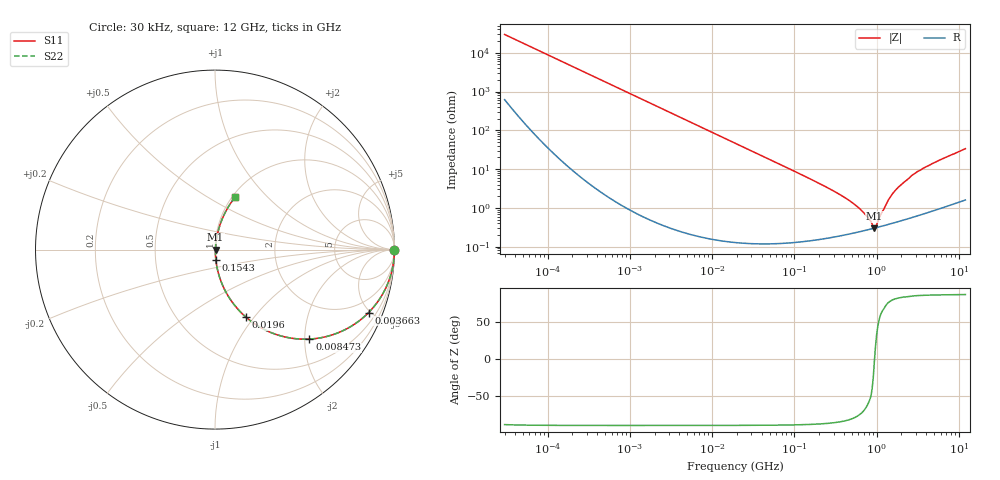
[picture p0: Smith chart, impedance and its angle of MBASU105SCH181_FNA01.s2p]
! MBASU105SCH181_FNA01  S-PARAMETER MODEL  ( General Type )
! Model Generated by TAIYO YUDEN Corporation (http://www.ty-top.com)
! Version 1.0
! TAIYO YUDEN Control No. 130207
! Copyright(c) 2013 TAIYO YUDEN CO.,LTD. All Rights Reserved.
! Product Description (link to TY-COMPAS)
! https://ds.yuden.co.jp/TYCOMPAS/or/detail?pn=MBASU105SCH181JFNA01&u=M
! Products Name : Multilayer Ceramic Capacitors
! Characteristics :
!  Capacitance : 180 pF , Rated Voltage : 50V , TCC : CH / C0H
!  Case Size : 1.0 x 0.5 / 0.039 x 0.02 [mm/inch] , Thickness : 0.5 / 0.02 [mm/inch]
!  (Conditions: Temperature = 25 degC , DC Bias Current/Voltage = 0A / 0V)
! External Node Assignments :
!  1  o---| |---o  2
! GND o---------o GND
! Frequency Range : 30000Hz  -  12GHz  [ 401 STEP ]
# MHz S RI R 50
! Freq[MHz].  S11 Real  S11 Imag  S21 Real  S21 Imag  S12 Real  S12 Imag  S22 Real  S22 Imag
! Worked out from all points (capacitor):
!   401 points, 30 kHz to 12 GHz, reference 50 ohm
!   read as one part in series: C = 178 pF near 32 kHz
!   lowest |Z| = 301 mohm at 939.2 MHz (marker M1)
!   series resonance near 943.3 MHz, so ESL is about 160 pH
!   S11 on the Smith chart (normalised r, x): 30 kHz: open; 3.663 MHz: 1.01, -4.87; 8.473 MHz: 1.00, -2.11; 19.6 MHz: 1.00, -0.91; 154.3 MHz: 1.00, -0.11; 12 GHz: 1.03, +0.67
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0.03  0.9999 -0.00336  8.15e-05 0.00336  8.15e-05 0.00336  0.9999 -0.00336
0.260295  0.9991 -0.0292  0.000901 0.0292  0.000901 0.0292  0.9991 -0.0292
0.886466  0.9901 -0.0984  0.00988 0.0984  0.00988 0.0984  0.9901 -0.0984
2.258455  0.9395 -0.2379  0.0605 0.2379  0.0605 0.2379  0.9395 -0.2379
3.663436  0.8554 -0.3512  0.1446 0.3512  0.1446 0.3512  0.8554 -0.3512
8.472713  0.5256 -0.4986  0.4744 0.4986  0.4744 0.4986  0.5256 -0.4986
12.08034  0.353 -0.4769  0.647 0.4769  0.647 0.4769  0.353 -0.4769
18.97367  0.1815 -0.3841  0.8185 0.3841  0.8185 0.3841  0.1815 -0.3841
19.5955  0.1722 -0.3762  0.8278 0.3762  0.8278 0.3762  0.1722 -0.3762
42.48934  0.0431 -0.2003  0.9569 0.2003  0.9569 0.2003  0.0431 -0.2003
154.3427  0.00458 -0.0562  0.9954 0.0562  0.9954 0.0562  0.00458 -0.0562
164.6252  0.00421 -0.0525  0.9958 0.0525  0.9958 0.0525  0.00421 -0.0525
324.0443  0.00243 -0.0248  0.9976 0.0248  0.9976 0.0248  0.00243 -0.0248
508.9517  0.00238 -0.0133  0.9976 0.0133  0.9976 0.0133  0.00238 -0.0133
702.6322  0.00263 -0.00688  0.9974 0.00688  0.9974 0.00688  0.00263 -0.00688
939.2353  0.003 -0.000145  0.997 0.000145  0.997 0.000145  0.003 -0.000145
1001.808  0.00311 0.00207  0.9969 -0.00207  0.9969 -0.00207  0.00311 0.00207
1428.372  0.00409 0.017  0.9959 -0.017  0.9959 -0.017  0.00409 0.017
1848.769  0.0056 0.034  0.9944 -0.034  0.9944 -0.034  0.0056 0.034
2998.885  0.0123 0.079  0.9877 -0.079  0.9877 -0.079  0.0123 0.079
5715.613  0.0359 0.1603  0.9641 -0.1603  0.9641 -0.1603  0.0359 0.1603
12000  0.1133 0.2941  0.8867 -0.2941  0.8867 -0.2941  0.1133 0.2941
